(* Logix 5000 AddOnInstructionDefinition export MSTL_Yaskawa; software revision 17.00 *)

TYPE Yaskawa_EIP_Servo :   // Yaskawa SigmaLogic Axis Structure v2.4.0
STRUCT
   O : Yaskawa_OUT_to_Servo;
   I : Yaskawa_IN_from_Servo;
   AOI_SB : Yaskawa_AOI_Status_Bits;
END_STRUCT
END_TYPE

TYPE Yaskawa_OUT_to_Servo :   // Structure of data sent out to the Yaskawa SigmaLogic controller v2.4.0
STRUCT
   b00_ServoOn : BOOL;   // Servo On
   b01_Stop : BOOL;   // Stops All Current Motion in Progress
   b02_Home : BOOL;   // Start Homing Process
   b03_MoveStart1 : BOOL;   // Start Current Motion
   b06_SuperImpose : BOOL;
   b07_ServoAlarmReset : BOOL;   // Servo Alarm Reset
   b08_ControllerAlarmReset : BOOL;   // SigmaLogic Alarm Reset
   b09_MoveStart2 : BOOL;   // Start Second Motion (Blended Move)
   b10_MoveAbort : BOOL;   // Abort Current Move
   b11_MovePause : BOOL;   // Pause Current Move
   b12_SeqPause : BOOL;   // Indexing Sequence Pause
   b13_SeqResume : BOOL;   // Indexing Sequence Resume
   b14_SeqCancel : BOOL;   // Indexing Sequence Cancel
   b15_AbsEncoderReset : BOOL;   // Absolute Encoder Reset
   b16_SeqStart : BOOL;   // Start Indexing Sequence
   b17_SeqEditSpeed : BOOL;   // Enter Edit Speed
   b18_SeqEditDistance : BOOL;   // Enter Distance Edit
   b19_PLSEnable : BOOL;   // Enable PLS execution
   b20_PLSActivateOutput1 : BOOL;   // Activate PLS output1 switch logic
   b21_PLSActivateOutput2 : BOOL;   // Activate PLS output2 switch logic
   b22_PLSActivateOutput3 : BOOL;   // Activate PLS output3 switch logic
   b23_PLSActivateOutput4 : BOOL;   // Activate PLS output4 switch logic
   b24_SetClock : BOOL;   // Set the remote controller clock with data provided by the PLC
   RebootController : BOOL;
   UseExternalEncoder : BOOL;   // Use External Encoder when executing MAHSP_Yaskawa
   b32_HeatbeatAnswer : BOOL;   // Heartbeat Answer
   BrakeBypassRequest : BOOL;
   SetFwdTorqueLimit : BOOL;
   SetRevTorqueLimit : BOOL;
   TorqueLimit : DINT;
   TorqueRamp : DINT;
   HomeMethod : INT;
   HomeSpeed : DINT;
   HomeAccDec : DINT;   // Home Move Acceleration/Deceleration Rate
   HomeBackOffDistance : DINT;
   HomeCreepSpeed : DINT;
   HomeCreepDistanceLimit : DINT;
   HomeCreepTimeLimit : DINT;
   HomeOffsetDistance : DINT;
   HomeOffsetSpeed : DINT;
   HomePostion : DINT;
   HomeTorque : DINT;
   HomeInputNo : DINT;
   HomeApproachTimeLimit : DINT;
   HomeApproachDistLimit : DINT;
   HomeDirection : INT;
   HomeSwitchMode : INT;
   MoveType : INT;
   MoveDirection : INT;
   MoveAccel1 : DINT;
   MoveAccel2 : DINT;
   MoveDecel1 : DINT;
   MoveDecel2 : DINT;
   MoveSpeed1 : DINT;
   MoveSpeed2 : DINT;
   MoveDistance1 : DINT;
   MoveDistance2 : DINT;
   MovePosition1 : DINT;
   MovePosition2 : DINT;
   RegistrationDistance : DINT;
   GearNumerator : DINT;
   GearDenominator : DINT;
   SuperImposeDistance : DINT;
   Resolution : INT;
   RegistrationDirection : INT;
   TuningLevel : INT;
   SequenceStep : INT;   // Staring Sequence Step Number
   SequenceEditStep : INT;   // Sequence Step Number to Edit
   FlagCommandBits1 : DINT;   // Flag Commands. 1..64 are General Flags, Bits 0..31 correspond to Flag 1..32
   FlagCommandBits2 : DINT;   // Flag Commands cont. 1..64 are General Flags, Bits 0..31 correspond to Flag 33..64
   DigitalOutCommandBits : DINT;   // Digital Output commands. Bits 0-7 correspond to CN13 Digital Outputs 0-7, used as Flag 73-80. Bits 8-10 correspond to CN1 Digital Outputs 0-2 used as Flag 88-90"
   SequenceEditSpeed : DINT;
   SequenceEditDistance : DINT;
   FeedRateOverride : INT;
   HSI_Enable : BOOL;
   HSI_MoveMode : BOOL;   // 0=Relative; 1=Moves per Cycle
   HSI_CalcMethod : BOOL;   // 0=Accel/Decel; 1=Time
   HSI_MoveDirection : BOOL;   // 0 = Negative; 1 = Positive
   HSI_TriggerFlag : INT;
   HSI_MovingFlag : INT;
   HSI_DwellingFlag : INT;
   HSI_DoneFlag : INT;
   HSI_MoveType : INT;   // 0=Single; 1=Repeat; 2=Repeat "x" times
   HSI_RepeatNumber : INT;
   HSI_Distance : DINT;
   HSI_Speed : DINT;
   HSI_Accel : DINT;
   HSI_MoveTime : DINT;
   HSI_DwellTime : DINT;
   PLS_OutputFlag1 : INT;
   PLS_OutputFlag2 : INT;
   PLS_OutputFlag3 : INT;
   PLS_OutputFlag4 : INT;
   PLS_OnPosition1 : DINT;
   PLS_OffPosition1 : DINT;
   PLS_OnPosition2 : DINT;
   PLS_OffPosition2 : DINT;
   PLS_OnPosition3 : DINT;
   PLS_OffPosition3 : DINT;
   PLS_OnPosition4 : DINT;
   PLS_OffPosition4 : DINT;
   PLS_OnCompensation1 : INT;
   PLS_OffCompensation1 : INT;
   PLS_OnCompensation2 : INT;
   PLS_OffCompensation2 : INT;
   PLS_OnCompensation3 : INT;
   PLS_OffCompensation3 : INT;
   PLS_OnCompensation4 : INT;
   PLS_OffCompensation4 : INT;
   RTC_Year : INT;
   RTC_Month : INT;
   RTC_Day : INT;
   RTC_Hour : INT;
   RTC_Min : INT;
   RTC_Sec : INT;
   StopDecel : DINT;
   AnalogOutput : INT;   // CN13, AO_01 [mV]
END_STRUCT
END_TYPE

TYPE Yaskawa_AOI_Status_Bits :   // Internal bits used to interlock Yaskawa AOI execution. v2.4.0
STRUCT
   MAM : BOOL;   // Move AOI Active
   MAJ : BOOL;   // Jog AOI Active
   MAB : BOOL;   // Blending AOI Active
   MAG : BOOL;   // Gearing AOI Active
   MAHSP : BOOL;   // Home SetPoint AOI Active
   MAH : BOOL;   // Homing AOI Active
   MSQE : BOOL;   // Sequence Edit AOI Active
   MSQR : BOOL;   // Sequence Run AOI Active
   MHSI : BOOL;   // High Speed Index AOI Active
   MSO : BOOL;   // Servo On
   MSF : BOOL;   // Servo Off
   MAFR : BOOL;   // Fault Reset
   MAS : BOOL;   // Servo Abort
   MTRQ : BOOL;   // Torque Mode Active
   MPLS : BOOL;   // PLS Active
   MCLK : BOOL;   // SetClock Active
   MSTL : BOOL;   // Set Torque Limit Active
   AOI_Permissive : BOOL;   // Permissive to Execute an AOI
END_STRUCT
END_TYPE

TYPE Yaskawa_IN_from_Servo :   // Structure of data coming from the Yaskawa SigmaLogic controller. v2.4.0
STRUCT
   AlarmText : STRING;   // ServoPack Alarm Code plus Text Description
   b00_Heartbeat : BOOL;
   b01_Alarm : BOOL;   // ServoPack Alarm
   b02_Warning : BOOL;   // ServoPack Warning
   b03_Ready : BOOL;   // ServoPack Ready
   b04_Enabled : BOOL;   // ServoPack Enabled ("Servo On")
   b05_StopComplete : BOOL;
   b06_HomeComplete : BOOL;
   b07_HomeBusy : BOOL;
   b08_HomeActive : BOOL;
   b09_HomeAborted : BOOL;
   b10_HomeError : BOOL;
   b11_MoveAbsComplete : BOOL;
   b12_MoveAbsBusy : BOOL;
   b13_MoveAbsActive : BOOL;
   b14_MoveAbsAborted : BOOL;
   b15_MoveAbsError : BOOL;
   b16_MoveRelComplete : BOOL;
   b17_MoveRelBusy : BOOL;
   b18_MoveRelActive : BOOL;
   b19_MoveRelAborted : BOOL;
   b20_MoveRelError : BOOL;
   b21_JogAtSpeed : BOOL;
   b22_JogBusy : BOOL;
   b23_JogActive : BOOL;
   b24_JogAborted : BOOL;
   b25_JogError : BOOL;
   b26_GearInSync : BOOL;
   b27_GearBusy : BOOL;
   b28_GearActive : BOOL;
   b29_GearAborted : BOOL;
   b30_GearError : BOOL;
   b32_MoveSuperComplete : BOOL;
   b33_MoveSuperBusy : BOOL;
   b34_MoveSuperActive : BOOL;
   b35_MoveSuperAborted : BOOL;
   b36_MoveSuperError : BOOL;
   b37_PowerCycleRequired : BOOL;
   b38_MoveBlend1Complete : BOOL;
   b39_MoveBlend1Busy : BOOL;
   b40_MoveBlend1Active : BOOL;
   b41_MoveBlend1Abort : BOOL;
   b42_MoveBlend1Error : BOOL;
   b43_MoveBlend2Complete : BOOL;
   b44_MoveBlend2Busy : BOOL;
   b45_MoveBlend2Active : BOOL;
   b46_MoveBlend2Abort : BOOL;
   b47_MoveBlend2Error : BOOL;
   b48_RegComplete : BOOL;
   b49_RegBusy : BOOL;
   b50_RegActive : BOOL;
   b51_RegAborted : BOOL;
   b52_RegError : BOOL;
   b53_ResetAbsEncoderActive : BOOL;
   b54_ResetAbsEncoderBusy : BOOL;
   b55_ResetAbsEncoderDone : BOOL;
   b56_ResetAbsEncoderError : BOOL;
   b57_SeqRunning : BOOL;
   b58_RegSensorNotReached : BOOL;
   b59_SeqEditError : BOOL;
   b60_SeqEditDone : BOOL;
   b61_TorqueAtTorque : BOOL;
   b62_TorqueBusy : BOOL;
   b63_TorqueActive : BOOL;
   b64_TorqueAborted : BOOL;
   b65_TorqueError : BOOL;
   b66_ControllerAlarm : BOOL;
   b67_ApplicationError : BOOL;
   b68_AxisAtStandStill : BOOL;
   b69_TestModeActive : BOOL;
   b70_ServoParamsOK : BOOL;
   b71_SetFwdTorqueLimitDone : BOOL;
   b72_SetRevTorqueLimitDone : BOOL;
   Position : DINT;
   Speed : DINT;
   Torque : DINT;
   HomeErrorID : INT;
   MoveAbsErrorID : INT;
   MoveRelErrorID : INT;
   JogErrorID : INT;
   GearErrorID : INT;
   MoveSuperErrorID : INT;
   ServoAlarmID : INT;
   ServoWarningID : INT;
   ControllerAlarmID : DINT;
   AxisGenAlarmID : DINT;
   MoveBlend1ErrorID : INT;
   MoveBlend2ErrorID : INT;
   ResetAbsEncoderErrorID : INT;
   FunctionBlockErrorID : INT;
   TorqueErrorID : INT;
   RegErrorID : INT;
   SeqCurrentStep : INT;
   FlagStatusBit1 : DINT;   // Flag Status. 1..64 are General Flags, Bits 0..31 correspond to Flag 1..32
   FlagStatusBit2 : DINT;   // Flag Status cont. 1..64 are General Flags, Bits 0..31 correspond to Flag 33..64
   IOStatusBits : DINT;   // Digital IO Status. Bits 0-7, CN13 Inputs 0-7, Used as Flag 65-72. Bits 8-15, CN13 Outputs 0-7, Used as Flag 73-80. Bits 16-22, CN1 Inputs 0-6, Used as Flag 81-87. Bits 23-25, CN1 Outputs 0-4, Used as Flag 88-92.
   HSI_Moving : BOOL;
   HSI_Dwelling : BOOL;
   HSI_Done : BOOL;
   HSI_Busy : BOOL;
   HSI_Error : BOOL;
   HSI_ErrorCode : INT;
   PLS_Running : BOOL;
   PLS_SwitchStatus1 : BOOL;
   PLS_SwitchStatus2 : BOOL;
   PLS_SwitchStatus3 : BOOL;
   PLS_SwitchStatus4 : BOOL;
   PLS_Busy : BOOL;
   PLS_Error : BOOL;
   PLS_ErrorCode : INT;
   SetClock_Done : BOOL;
   SetClock_Busy : BOOL;
   SetClock_Error : BOOL;
   SetClock_ErrorID : INT;
   SoftwareVersion : DINT;
   FirmwareVersion : DINT;
   CommandedPos : DINT;
   CommandedPosNonCyc : DINT;
   CommandedSpeed : DINT;
   Clock_Year : INT;
   Clock_Month : INT;
   Clock_Day : INT;
   Clock_Hour : INT;
   Clock_Minute : INT;
   Clock_Second : INT;
   AnalogInput : REAL;   // CN13, AI_01 [v]
   BrakeBypassActive : BOOL;
   ForwardTorqueLimit : DINT;
   ReverseTorqueLimit : DINT;
END_STRUCT
END_TYPE

ADD_ON_INSTRUCTION MSTL_Yaskawa   (* revision 2.4 0, vendor Yaskawa America, Inc., ExecuteEnableInFalse *)
// Motion Set Torque Limit
// Revision note:
// 2.4.0: Updated AOI  help description.
// 2.3.1: Moved unlatch of AOI_ON_LOCAL to bottom of EnableInFalse routine so that outputs will be on for at least 1 scan if one-shot on EN is used.
// 2.3.0: Initial Release 12/20/2018
// Help:
// Sets a Torque or Force limit on the axis in either the Forward or Reverse direction. Both forward and reverse limits can be applied at the same time but there is only a single input for the limit setting. In this case, both Forward and Reverse limits would set to the same value.
// This AOI can operate simultaneously with nearly all other AOI's except the Homing AOI's (MAH and MAHSP). In this case, FLT_BSY will be set.
// Value for torque/force limit should always be a positive number with valid range of 0-800 % of motors rated torque/force. The limits can be set during motion.
VAR_IN_OUT
   Axis : Yaskawa_EIP_Servo; {required}
END_VAR
VAR_INPUT
   SetForwardLimit : INT; {required}   // 0: Do not set to new value 1: Set to new value
   SetReverseLimit : INT; {required}   // 0: Do not set to new value 1: Set to new value
   TorqueLimit : DINT; {required}   // Torque/Force Limit Setting Valid range: 0-800% of rated motor torque/force
END_VAR
VAR_OUTPUT
   EN : BOOL; {visible}   // Function is Executing
   DN : BOOL; {visible}   // Servo Torque/Force Limit parameter has been sent
   FLT_PRM : BOOL; {visible}   // Invalid Parameter
   FLT_BSY : BOOL; {visible}   // There is another AOI Active for this Axis [MAH or MAHSP]
END_VAR
VAR
   AOI_ON_LOCAL : BOOL;
   Finished : BOOL;   // Function is Finished
END_VAR

ROUTINE EnableInFalse   (* ladder *)
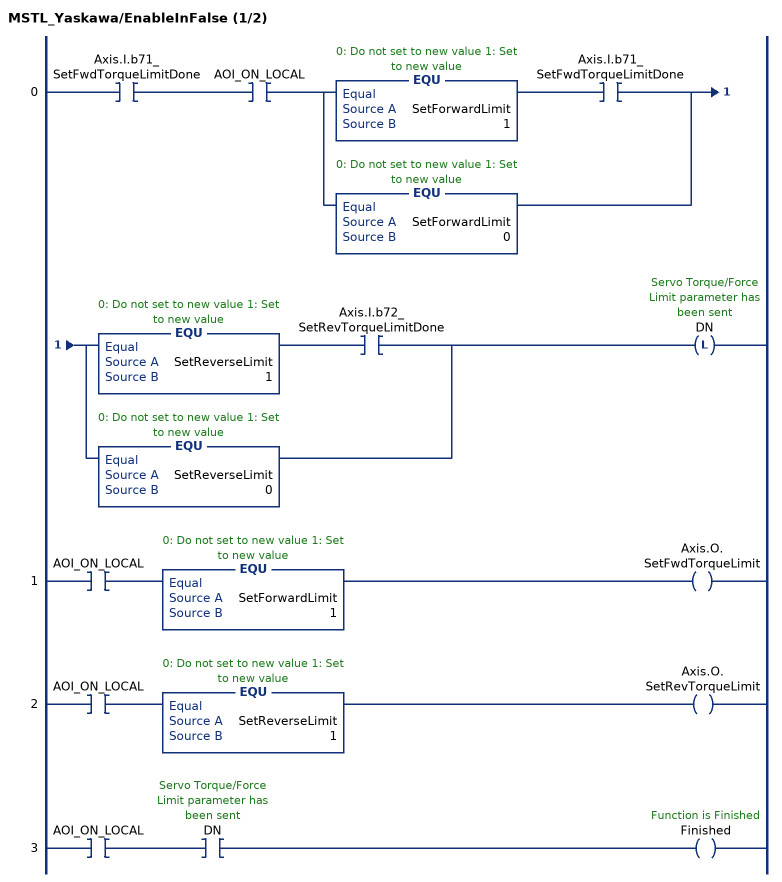
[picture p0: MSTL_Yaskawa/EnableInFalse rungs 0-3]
   0: XIC(Axis.I.b71_SetFwdTorqueLimitDone)XIC(AOI_ON_LOCAL)[EQU(SetForwardLimit,1) XIC(Axis.I.b71_SetFwdTorqueLimitDone) ,EQU(SetForwardLimit,0) ][EQU(SetReverseLimit,1) XIC(Axis.I.b72_SetRevTorqueLimitDone) ,EQU(SetReverseLimit,0) ]OTL(DN);
   1: XIC(AOI_ON_LOCAL)EQU(SetForwardLimit,1)OTE(Axis.O.SetFwdTorqueLimit);
   2: XIC(AOI_ON_LOCAL)EQU(SetReverseLimit,1)OTE(Axis.O.SetRevTorqueLimit);
   3: XIC(AOI_ON_LOCAL)XIC(DN)OTE(Finished);
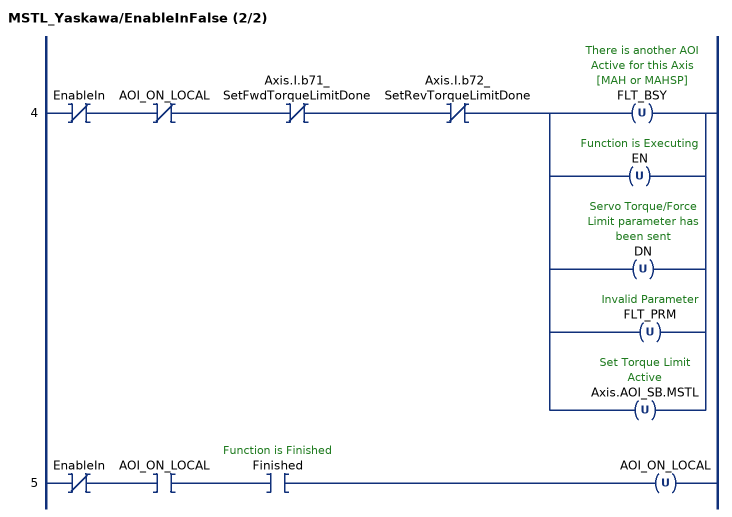
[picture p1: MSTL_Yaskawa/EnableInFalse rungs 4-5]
   4: XIO(EnableIn)XIO(AOI_ON_LOCAL)XIO(Axis.I.b71_SetFwdTorqueLimitDone)XIO(Axis.I.b72_SetRevTorqueLimitDone)[OTU(FLT_BSY) ,OTU(EN) ,OTU(DN) ,OTU(FLT_PRM) ,OTU(Axis.AOI_SB.MSTL) ];
   5: XIO(EnableIn)XIC(AOI_ON_LOCAL)XIC(Finished)OTU(AOI_ON_LOCAL);
END_ROUTINE

ROUTINE Logic   (* ladder *)
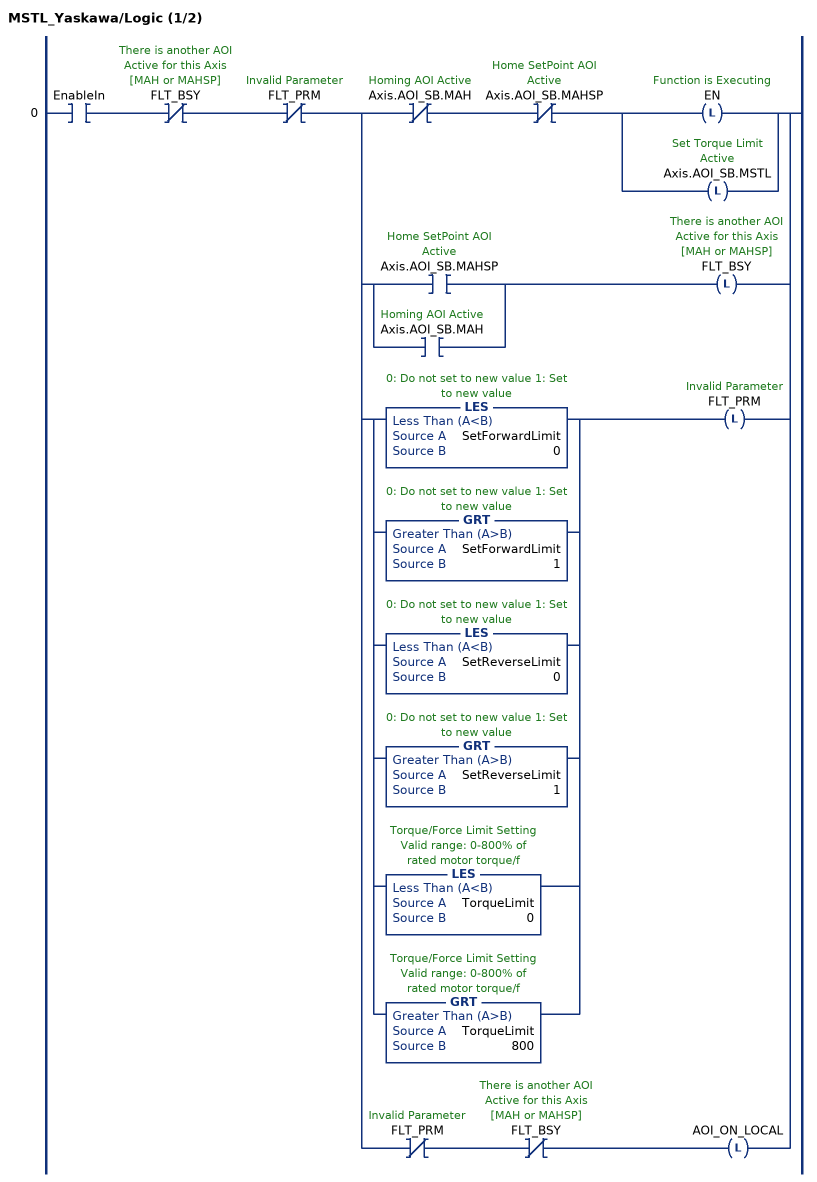
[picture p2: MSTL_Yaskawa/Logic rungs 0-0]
   0: XIC(EnableIn)XIO(FLT_BSY)XIO(FLT_PRM)[XIO(Axis.AOI_SB.MAH) XIO(Axis.AOI_SB.MAHSP) [OTL(EN) ,OTL(Axis.AOI_SB.MSTL) ] ,[XIC(Axis.AOI_SB.MAHSP) ,XIC(Axis.AOI_SB.MAH) ] OTL(FLT_BSY) ,[LES(SetForwardLimit,0) ,GRT(SetForwardLimit,1) ,LES(SetReverseLimit,0) ,GRT(SetReverseLimit,1) ,LES(TorqueLimit,0) ,GRT(TorqueLimit,800) ] OTL(FLT_PRM) ,XIO(FLT_PRM) XIO(FLT_BSY) OTL(AOI_ON_LOCAL) ];
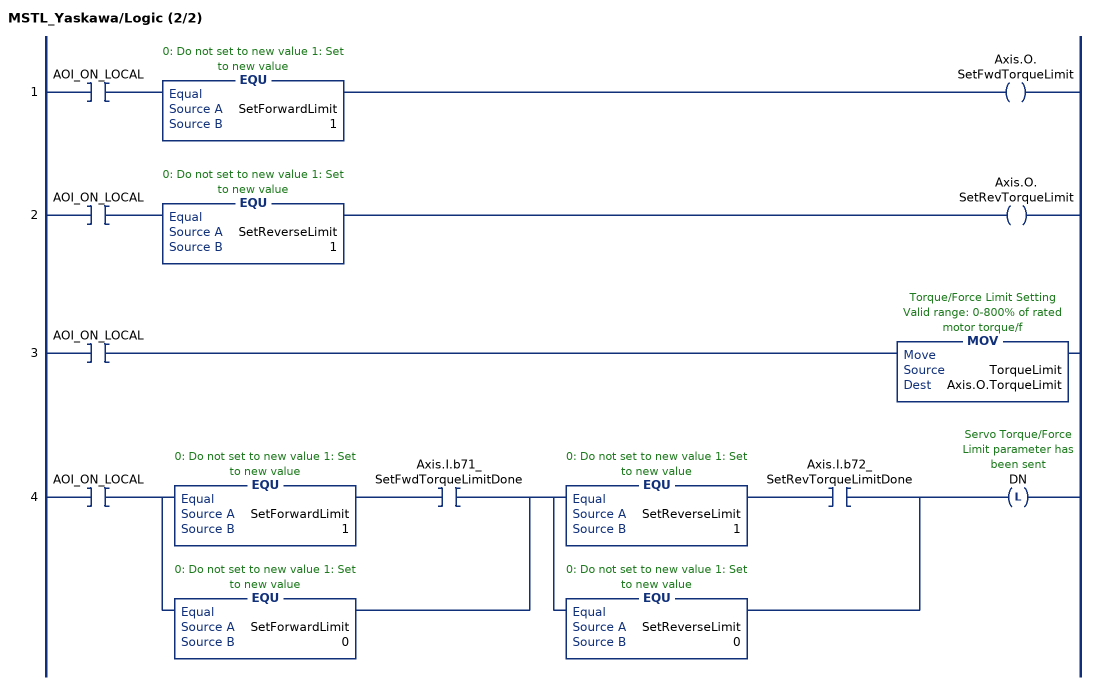
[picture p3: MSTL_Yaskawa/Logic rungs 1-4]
   1: XIC(AOI_ON_LOCAL)EQU(SetForwardLimit,1)OTE(Axis.O.SetFwdTorqueLimit);
   2: XIC(AOI_ON_LOCAL)EQU(SetReverseLimit,1)OTE(Axis.O.SetRevTorqueLimit);
   3: XIC(AOI_ON_LOCAL)MOV(TorqueLimit,Axis.O.TorqueLimit);
   4: XIC(AOI_ON_LOCAL)[EQU(SetForwardLimit,1) XIC(Axis.I.b71_SetFwdTorqueLimitDone) ,EQU(SetForwardLimit,0) ][EQU(SetReverseLimit,1) XIC(Axis.I.b72_SetRevTorqueLimitDone) ,EQU(SetReverseLimit,0) ]OTL(DN);
END_ROUTINE
END_ADD_ON_INSTRUCTION
